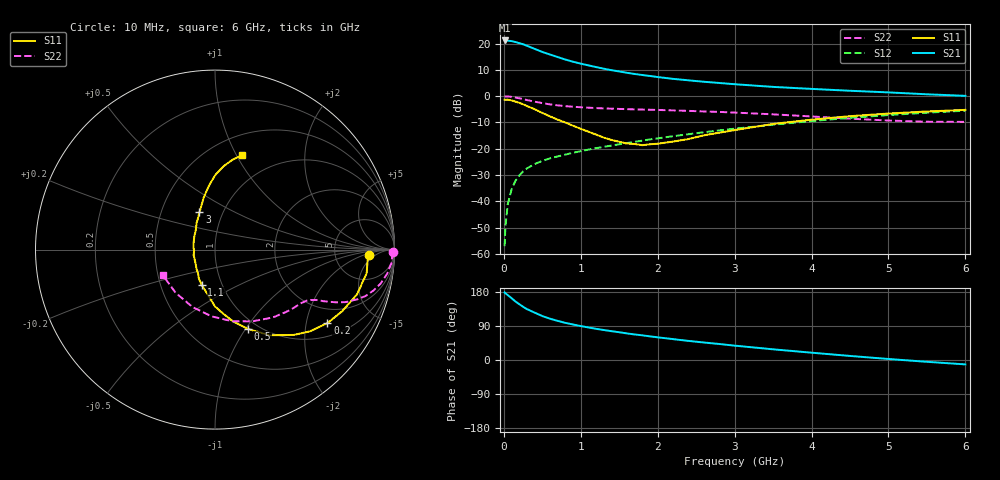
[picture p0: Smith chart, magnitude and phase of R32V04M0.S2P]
! SIEMENS Small Signal Semiconductors
! BFR181
! Si NPN RF Bipolar Junction Transistor in SOT23
! VCE = 2 V  IC = 4 mA
! Common Emitter S-Parameters:  May  1996
# GHz  S  MA  R  50
!  f  S11  S21  S12  S22
! GHz  MAG  ANG  MAG  ANG  MAG  ANG  MAG  ANG
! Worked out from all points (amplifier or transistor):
!   36 points, 10 MHz to 6 GHz, reference 50 ohm
!   highest |S21| = 21.2 dB at 10 MHz (marker M1)
!   |S21| within 3 dB of that: start of sweep to 383.1 MHz
!   unconditionally stable (mu >= 1): 1.203 GHz to 3.064 GHz
!   at 250 MHz: K = 0.37, MSG = 24.2 dB, |S12| = -28.6 dB
!   at 1.4 GHz: K = 1.05, MAG = 13.0 dB, |S12| = -18.8 dB
!   at 6 GHz: K = 0.86, MSG = 2.8 dB, |S12| = -5.5 dB
!   S11 on the Smith chart (normalised r, x): 10 MHz: 13, -3; 200 MHz: 1.43, -2.66; 500 MHz: 0.90, -1.03; 1.1 GHz: 0.80, -0.33; 3 GHz: 0.78, +0.34; 6 GHz: 0.70, +1.06
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0.01  0.8583 -1.9  11.46 178.3  0.0014 95.7  0.9935 -0.9
0.02  0.8525 -3.5  11.44 176.3  0.0032 92.5  0.9874 -1.7
0.05  0.8551 -8.8  11.36 171.4  0.0087 84.6  0.9873 -4.1
0.1  0.8301 -17.4  11.14 163.3  0.0167 81.5  0.9685 -8.0
0.15  0.7876 -25.8  10.7 154.5  0.0244 75.0  0.942 -11.6
0.2  0.7484 -33.2  10.2 147.5  0.0309 72.9  0.9116 -14.5
0.25  0.6981 -40.7  9.701 140.4  0.037 69.2  0.8783 -17.1
0.3  0.6478 -47.2  9.081 134.3  0.0423 67.3  0.8429 -19.1
0.4  0.5652 -57.6  7.927 125.0  0.0511 63.6  0.7844 -21.9
0.5  0.4794 -67.3  6.923 116.0  0.0586 61.7  0.737 -23.5
0.6  0.4124 -75.9  6.188 109.0  0.0655 60.8  0.6972 -24.6
0.7  0.3567 -83.2  5.539 103.2  0.0714 60.6  0.6673 -25.5
0.8  0.3152 -90.2  4.96 98.0  0.0773 60.4  0.6446 -26.0
0.9  0.2735 -95.7  4.507 93.6  0.0837 60.3  0.6285 -26.5
1.1  0.2105 -110.6  3.844 85.8  0.0961 61.1  0.6027 -27.8
1.6  0.1255 -155.0  2.777 70.1  0.1283 62.0  0.5654 -31.8
2.2  0.1366 147.5  2.13 55.1  0.1731 61.2  0.5355 -39.0
3  0.2258 112.5  1.685 37.9  0.2403 57.4  0.4868 -51.7
3.5  0.2957 102.3  1.499 28.2  0.2864 53.5  0.4504 -62.6
4.5  0.4155 89.8  1.265 10.7  0.3865 43.5  0.3728 -92.8
5.5  0.5105 78.9  1.084 -4.8  0.4844 30.7  0.3256 -132.5
6  0.5481 73.8  1.013 -11.6  0.5291 23.6  0.3242 -154.0
